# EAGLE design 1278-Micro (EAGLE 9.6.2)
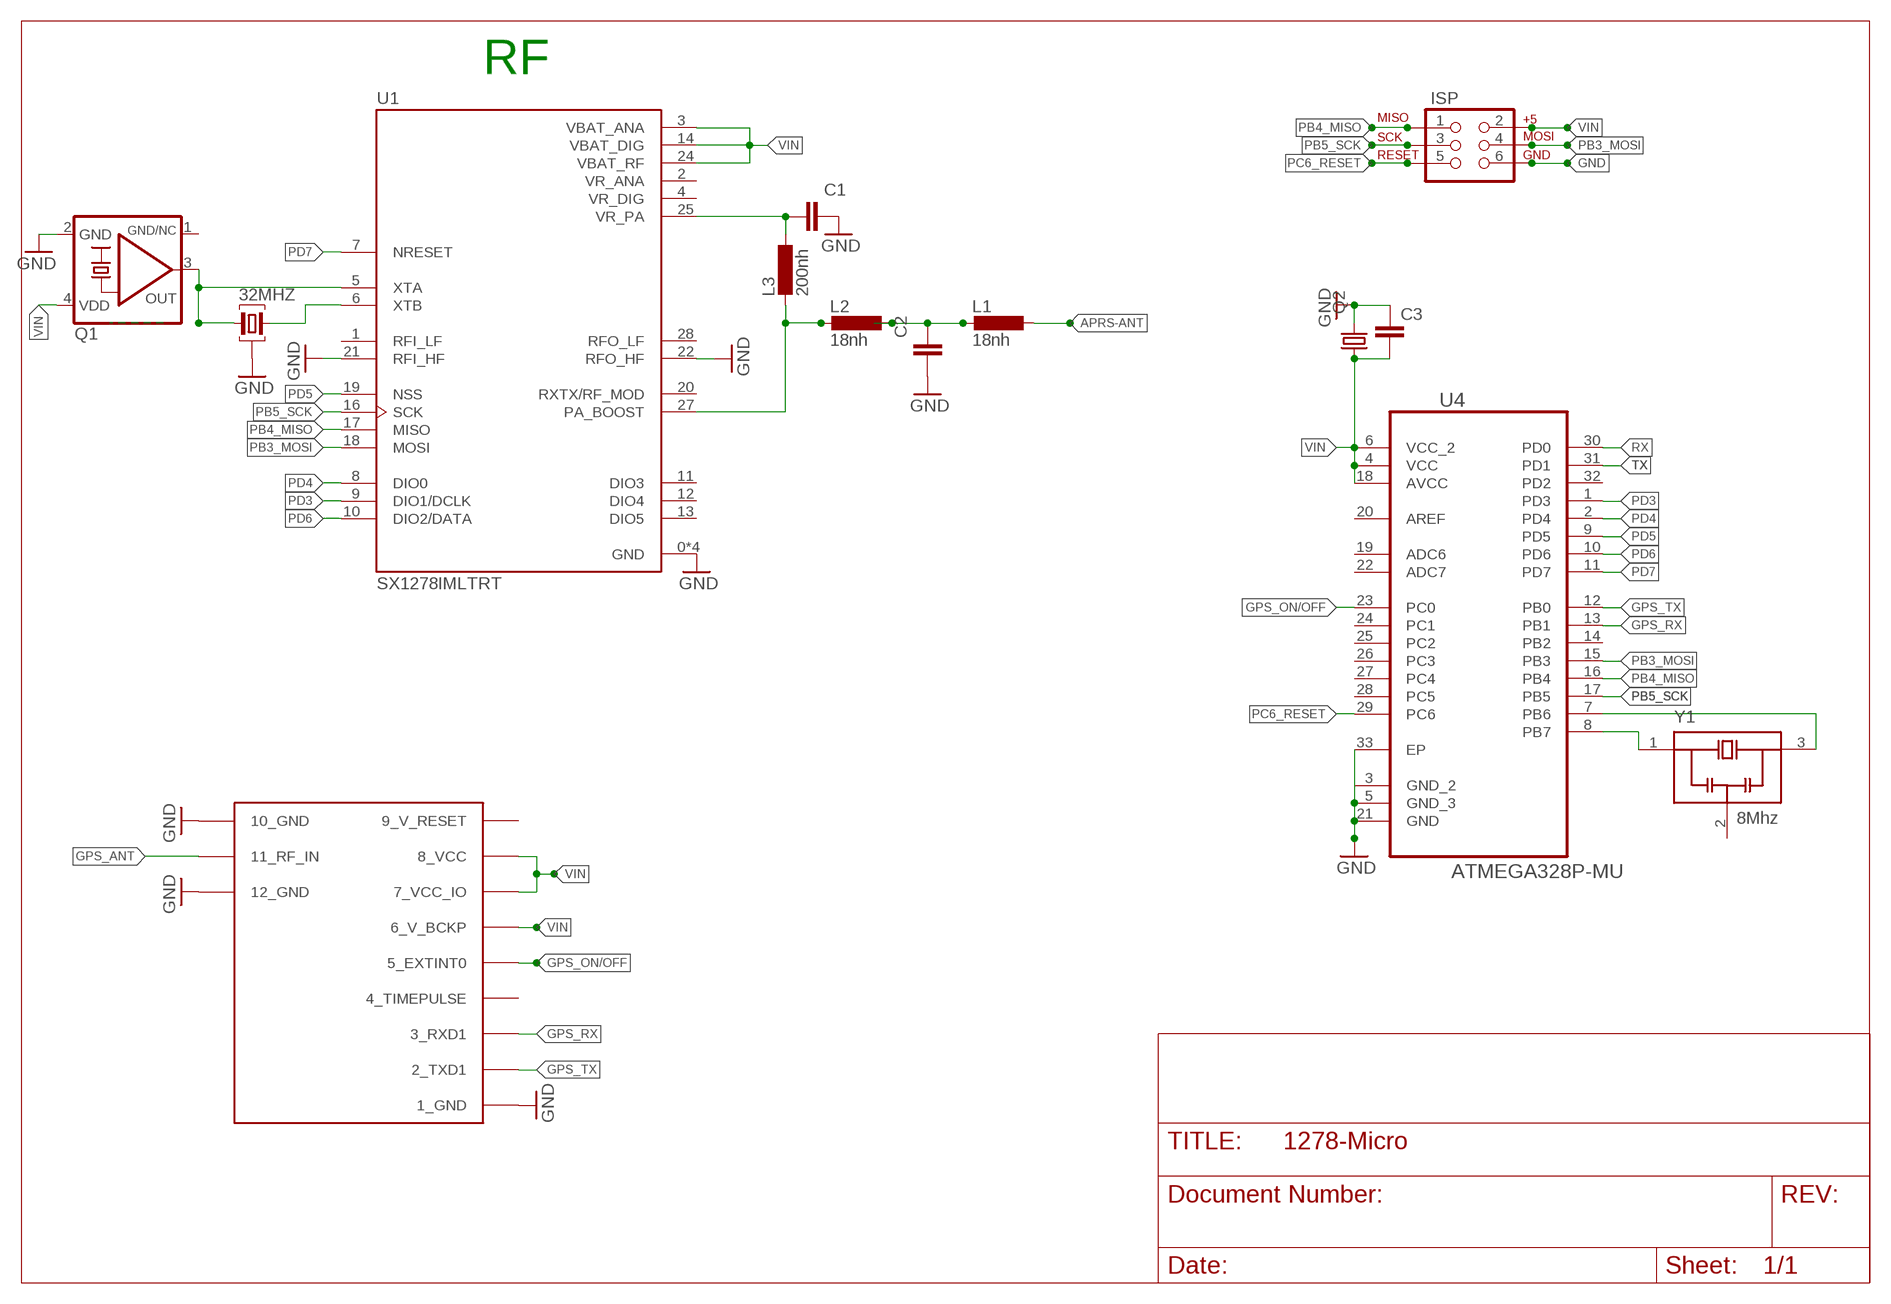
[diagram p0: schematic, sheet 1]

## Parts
32MHZ  16Mhz  ABM8G  [ABM8G]
C1  100nF  C-EUC0603K  [C0603K]
C2  15pF  C-EUC0603K  [C0603K]
C3  C-EUC1808  [C1808]
ISP  AVR_SPI_PRG_6PTH  [2X3]
L1  18nh  L-EUL2012C  [L2012C]
L2  18nh  L-EUL2012C  [L2012C]
L3  200nh  L-EUL2012C  [L2012C]
Q1  TCXO 32Mhz  KXO-TCXO-CMOS-84  [3.2X2.5_KXO-84-TCXO]
Q2  KX-327-NHF  [3.2X1.5]
U1  SX1278IMLTRT  [QFN65P600X600X100-29N]
U4  ATMEGA328P-MU  [QFN50P500X500X100-33N]
U$2  UBLOX_MAX  [UBLOX_MAX]
Y1  8Mhz  CSTCE12M0G15L08-R0  [OSC_CSTCE12M0G15L08-R0]

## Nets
AAA: 32MHZ.1 Q1.3(OUT) U1.5(XTA)
APRS-ANT: L1.1
GND: 32MHZ.2 32MHZ.4 C1.2 C2.1 C3.1 ISP.6 Q1.2(GND) Q2.2 U1.0(GND) U1.15(GND) U1.21(RFI_HF) U1.22(RFO_HF) U1.23(GND) U1.26(GND) U4.3(GND_2) U4.5(GND_3) U4.21(GND) U4.33(EP) U$2.1_GND U$2.10_GND U$2.12_GND
GPS_ANT: U$2.11_RF_IN
GPS_ON/OFF: U4.23(PC0) U$2.5_EXTINT0
GPS_RX: U4.13(PB1) U$2.3_RXD1
GPS_TX: U4.12(PB0) U$2.2_TXD1
N$1: U4.7(PB6) Y1.3(OUT)
N$2: U4.8(PB7) Y1.1(IN)
N$3: C2.2 L1.2 L2.1
N$8: C1.1 L3.1 U1.25(VR_PA)
N$9: L2.2 L3.2 U1.27(PA_BOOST)
N$15: 32MHZ.3 U1.6(XTB)
PB3_MOSI: ISP.4 U1.18(MOSI) U4.15(PB3)
PB4_MISO: ISP.1 U1.17(MISO) U4.16(PB4)
PB5_SCK: ISP.3 U1.16(SCK) U4.17(PB5)
PC6_RESET: ISP.5 U4.29(PC6)
PD3: U1.9(DIO1/DCLK) U4.1(PD3)
PD4: U1.8(DIO0) U4.2(PD4)
PD5: U1.19(NSS) U4.9(PD5)
PD6: U1.10(DIO2/DATA) U4.10(PD6)
PD7: U1.7(NRESET) U4.11(PD7)
RX: U4.30(PD0)
TX: U4.31(PD1)
VIN: C3.2 ISP.2 Q1.4(VDD) Q2.1 U1.3(VBAT_ANA) U1.14(VBAT_DIG) U1.24(VBAT_RF) U4.4(VCC) U4.6(VCC_2) U4.18(AVCC) U$2.6_V_BCKP U$2.7_VCC_IO U$2.8_VCC
Unconnected: U1.1(RFI_LF) U1.11(DIO3) U1.12(DIO4) U1.13(DIO5) U1.20(RXTX/RF_MOD) U1.28(RFO_LF) U4.14(PB2) U4.19(ADC6) U4.20(AREF) U4.22(ADC7) U4.24(PC1) U4.25(PC2) U4.26(PC3) U4.27(PC4) U4.28(PC5) U4.32(PD2) U$2.4_TIMEPULSE

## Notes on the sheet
- RF

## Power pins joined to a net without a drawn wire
9_V_RESET: U$2.9_V_RESET
GND: Y1.2(GND)
GND/NC: Q1.1(GND/NC)
VR_ANA: U1.2(VR_ANA)
VR_DIG: U1.4(VR_DIG)

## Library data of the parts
32MHZ = crystal:ABM8G: CRYSTAL - ABRACON ABM8G Series, 3.2 x 2.5 mm
C1 C2 = rcl:C-EU: CAPACITOR, European symbol; SPICEPREFIX: C
C3 = resistor:C-EU: CAPACITOR, European symbol
ISP = SparkFun:AVR_SPI_PRG_6: AVR ISP 6 Pin This is the reduced ISP connector for AVR programming. Common on Arduino. This footprint will take up less PCB space and can be used with a 10-pin to 6-pin adapter such as SKU: BOB-08508
L1-L3 = resistor:L-EU: INDUCTOR, European symbol
Q1 = crystal-geyer_V1_0:KXO-TCXO-CMOS: TCXO : CMOS - Serie Model Size l/w/h [mm] Frequency Range Frequency Stability Temp. Range [°C] Output AECQ 200 availabel Datasheet KXO-86 KXO-84 KXO-83 KXO-82 2.5/2.0/0.7 3.2/2.5/1.0 5.0/3.2/1.5 7.0/5.0/2.4 13,0 ~ 40,0 MHz 10,0 ~ 40,0 MHz 10,0 ~ 40,0 MHz 10,0 ~ 30,0 MHz ±1,0 … ±2,5ppm ±1,0 …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
Q2 = crystal-geyer_V1_0:KX-327
U1 = SX1278IMLTRT:SX1278IMLTRT; DESCRIPTION: IC RF TxRx Only 802.15.4 LoRa™ 137MHz ~ 525MHz 28-VQFN Exposed Pad; DIGI-KEY_PART_NUMBER: SX1278IMLTRTCT-ND; MF: Semtech; MP: SX1278IMLTRT; PACKAGE: VQFN-28 Semtech
U4 = ava:ATMEGA328P-MU: Programmable Flash; MPN: ATMEGA328P-MU; OC_FARNELL: 1748522; OC_NEWARK: 26R2526; PACKAGE: QFN-32; SUPPLIER: Atmel
U$2 = Max gps:UBLOX_MAX: UBLOX MAX
Y1 = CSTCE12M0G15L08-R0:CSTCE12M0G15L08-R0: 8MHz Ceramic Resonator Built in Capacitor 10pF +/- 0.2% -40C - 125C Surface Mount Check prices; AVAILABILITY: Not in stock; DESCRIPTION: CSTCE Series 12 MHz 3.2 x 1.3 x 0.7 mm Built-in Capacitor SMT Resonator; MF: Murata; MP: CSTCE12M0G15L08-R0; PACKAGE: SMD-3 Murata; PRICE: None

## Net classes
0 default: width 0.203 mm
1 vcc: width 0.152 mm, clearance 0.152 mm

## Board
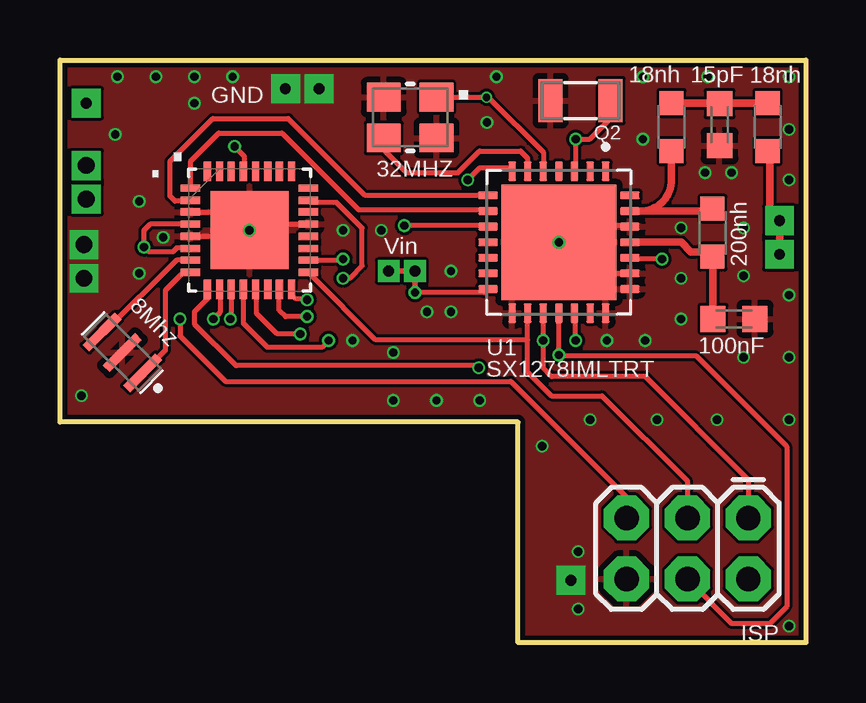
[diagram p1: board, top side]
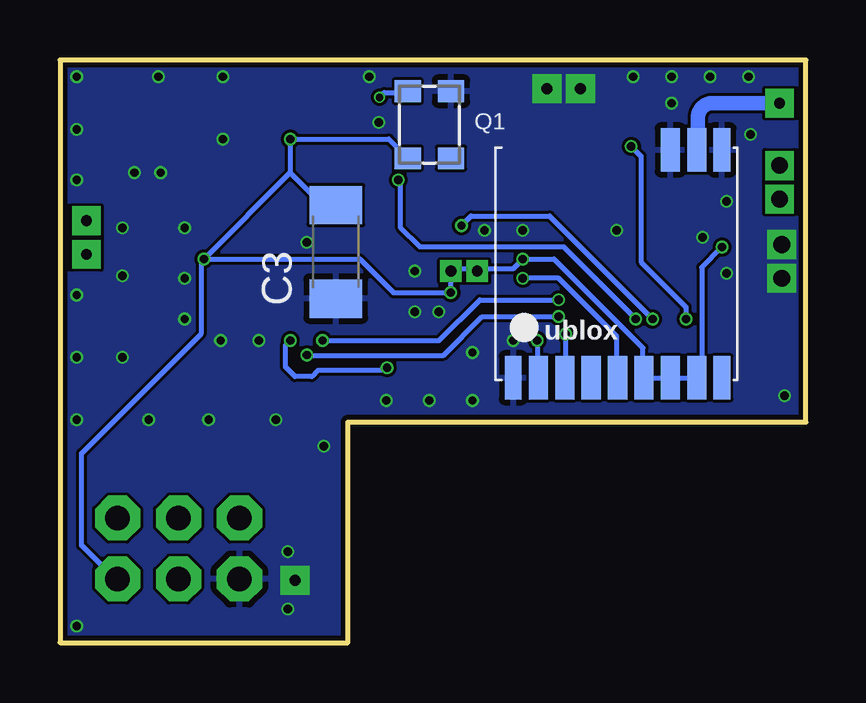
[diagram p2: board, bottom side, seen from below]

Size 31.1 x 24.3 mm. Coordinates in mm from the lower left corner, seen from the top.
Outline: 0,24.3 31.1,24.3 31.1,0 19.1,0 19.1,9.2 0,9.2 0,24.3
Copper layers (1*16): Top 0.035559375mm / dielectric 1.6mm / Bottom 0.035559375mm
Design rules "jlcpcb2layer *": minimum track width 5mil, minimum drill 12mil, track to track 5mil, track to pad 5mil, pad to pad 5mil, via to via 5mil, smd to smd 5mil, copper to edge 8mil, drill to drill 6mil, minimum pad ring 5mil, minimum via ring 3mil, stop-mask expansion 2.5mil, vias tented up to drill 14mil, thermal gap 10mil

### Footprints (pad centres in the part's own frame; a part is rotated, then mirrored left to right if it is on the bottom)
ABM8G = smd 1.4 x 1.2: 1 -1.1,-0.85; 2 1.1,-0.85; 3 1.1,0.85; 4 -1.1,0.85
C0603K = smd 1.05 x 1.08: 1 -0.875,0; 2 0.875,0
C1808 = smd 1.6 x 2.2: 1 -1.95,0; 2 1.95,0
2X3 = drill 1.016 pad 1.88 octagon: 1 0,0; 2 0,2.54; 3 2.54,0; 4 2.54,2.54; 5 5.08,0; 6 5.08,2.54
L2012C = smd 1 x 1: 1 -1,0; 2 1,0
3.2X2.5_KXO-84-TCXO = smd 0.9 x 1.1: 1 -1.4,-0.9; 2 1.4,-0.9; 3 1.4,0.9; 4 -1.4,0.9
3.2X1.5 = smd 1 x 1.8: 1 -1.25,0; 2 1.25,0
QFN65P600X600X100-29N = smd 4.8 x 4.8: 0 0,0 | smd 0.81 x 0.32: 1 -2.955,1.95; 2 -2.955,1.3; 3 -2.955,0.65; 4 -2.955,0; 5 -2.955,-0.65; 6 -2.955,-1.3; 7 -2.955,-1.95; 15 2.955,-1.95; 16 2.955,-1.3; 17 2.955,-0.65; 18 2.955,0; 19 2.955,0.65; 20 2.955,1.3; 21 2.955,1.95 | smd 0.32 x 0.81: 8 -1.95,-2.955; 9 -1.3,-2.955; 10 -0.65,-2.955; 11 0,-2.955; 12 0.65,-2.955; 13 1.3,-2.955; 14 1.95,-2.955; 22 1.95,2.955; 23 1.3,2.955; 24 0.65,2.955; 25 0,2.955; 26 -0.65,2.955; 27 -1.3,2.955; 28 -1.95,2.955
QFN50P500X500X100-33N = smd 0.813 x 0.305: 1 -2.464,1.753; 2 -2.464,1.245; 3 -2.464,0.762; 4 -2.464,0.254; 5 -2.464,-0.254; 6 -2.464,-0.762; 7 -2.464,-1.245; 8 -2.464,-1.753; 17 2.464,-1.753; 18 2.464,-1.245; 19 2.464,-0.762; 20 2.464,-0.254; 21 2.464,0.254; 22 2.464,0.762; 23 2.464,1.245; 24 2.464,1.753 | smd 0.305 x 0.813: 9 -1.753,-2.464; 10 -1.245,-2.464; 11 -0.762,-2.464; 12 -0.254,-2.464; 13 0.254,-2.464; 14 0.762,-2.464; 15 1.245,-2.464; 16 1.753,-2.464; 25 1.753,2.464; 26 1.245,2.464; 27 0.762,2.464; 28 0.254,2.464; 29 -0.254,2.464; 30 -0.762,2.464; 31 -1.245,2.464; 32 -1.753,2.464 | smd 3.251 x 3.251: 33 0,0
UBLOX_MAX = smd 1.8 x 0.7: 1_GND 4.95,-4.4; 9_V_RESET 4.95,4.3; 10_GND -4.55,4.3 | smd 1.8 x 0.8: 2_TXD1 4.95,-3.35; 3_RXD1 4.95,-2.25; 4_TIMEPULSE 4.95,-1.15; 5_EXTINT0 4.95,-0.05; 6_V_BCKP 4.95,1.05; 7_VCC_IO 4.95,2.15; 8_VCC 4.95,3.25; 11_RF_IN -4.55,3.25; 12_GND -4.55,2.15
OSC_CSTCE12M0G15L08-R0 = smd 0.4 x 1.9: 1 -1.2,0; 2 0,0; 3 1.2,0

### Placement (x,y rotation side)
32MHZ  14.6,21.9 180 top
C1  28.1,13.5 0 top
C2  27.5,21.6 90 top
C3  19.6,16.3 90 bottom
ISP  28.7,5.2 180 top
L1  29.5,21.5 90 top
L2  25.5,21.5 270 top
L3  27.2,17.1 90 top
Q1  15.7,21.6 90 bottom
Q2  21.7,22.6 180 top
U1  20.8,16.7 270 top
U4  7.9,17.2 0 top
U$2  7.8,16 270 bottom
Y1  2.6,12.1 135 top

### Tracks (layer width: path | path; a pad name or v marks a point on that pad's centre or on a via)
AAA  (via drill 0.3)
  Top 0.203: 32MHZ.1 v17.78,22.75 | v17.78,22.75 17.85,22.75 20.15,20.45 U1.5 | v17.78,22.74 v17.78,22.75
  Bottom 0.203: v17.78,22.74 17.58,22.94 16.66,22.94 Q1.3
APRS-ANT  (via drill 0.45 pad 1.2)
  Top 0.305: v30,16.2 v30,17.6 arc-90 29.6,18 29.6,20.4 L1.1
GND  (via drill 0.35, 0.45 pad 1.2, 0.7 pad 1.2)
  Top 0.203: U4.5 6.75,16.95 6.8,16.9 7.1,16.9 | 7.1,16.9 7.89,16.9 | 7.89,16.9 8.6,16.9 9.15,17.45 U4.21 | U4.3 6.74,17.96 7.1,17.6 7.1,16.9 | 7.89,16.9 7.89,17.14 U4.33 | 22.2,17.29 21.3,17.29 20.84,16.84 U1.0 | U1.26 23.71,17.39 22.2,17.39 22.2,17.29 | U1.23 22.6,15.4 22.2,15.8 22.2,17.29
  other vias: 13.9,12.1 15.3,13.8 21.6,1.4 4.3,16.9 13.9,10.1 1,16.6 1,15.2 2.3,21.2 2.4,23.6 7.2,23.6 15.7,10.1 17.5,10.1 21.6,3.8 30.4,0.7 3.3,18.4 17.8,21.7 18.2,23.6 27,23.6 30.4,23.6 24.4,12.6 22.8,12.6 30.4,19.3 30.4,21.4 28,19.6 26.9,19.6 24.3,21 25.9,17.3 25.9,13.5 28.5,17.3 28.5,15.3 30.4,14.5 30.4,11.9 28.5,11.9 25.9,15.2 12.2,12.6 22.1,9.3 24.9,9.3 27.4,9.3 20.1,8.2 16.3,13.8 5.6,23.6 4,23.6 5.6,22.5 20.8,16.7 11.8,17.2 13.4,17.2 30.4,9.3 10.8,23.1 9.4,23.1 16.3,15.5 0.9,10.3 3.3,15.4 24.3,23.6 7.9,17.2 21.3,2.6
  pour Top: -12.19,36.02 41.75,36.02 41.75,-7.09 -12.19,-7.09
  pour Bottom: -12.19,36.02 41.75,36.02 41.75,-7.09 -12.19,-7.09
GPS_ANT  (via drill 0.45 pad 1.2)
  Bottom 0.203: 4.5,20.6 arc90 U$2.11_RF_IN
  Bottom 0.61: v1.1,22.5 3.9,22.5 arc-90 4.5,21.9 4.5,20.6
GPS_ON/OFF  (via drill 0.35)
  Top 0.203: U4.23 10.45,18.36 11.54,18.36 12.6,17.29 12.6,15.72 12.09,15.2 v11.8,15.2
  Bottom 0.203: v11.8,15.2 10.31,15.2 7.89,12.77 7.89,11.2 U$2.5_EXTINT0
GPS_RX  (via drill 0.35)
  Top 0.203: v10.02,12.87 9.06,12.87 8.19,13.74 8.19,14.7 U4.13
  Bottom 0.203: U$2.3_RXD1 10.02,11.08 v10.02,12.87
GPS_TX  (via drill 0.35)
  Top 0.203: U4.12 7.64,14.73 7.64,13.34 8.66,12.32 10.92,12.32 v11.2,12.6
  Bottom 0.203: v11.2,12.6 v11.19,12.59 11.19,11.09 U$2.2_TXD1
N$1
  Top 0.203: U4.7 4.86,15.96 1.85,12.95 Y1.3
N$2
  Top 0.203: Y1.1 4.4,12.2 4.4,14.7 5.15,15.45 U4.8
N$3
  Top 0.203: 27.15,22.5 27.18,22.48 C2.2 27.53,22.5
  Top 0.305: L2.1 27.15,22.5 | L1.2 27.53,22.5
N$8
  Top 0.203: L3.1 27.22,16.07
  Top 0.305: U1.25 25.9,16.7 26.3,16.3 27,16.3 L3.1 | 27.22,16.07 C1.1
N$9
  Top 0.203: L3.2 27.25,18.1 27.35,18
  Top 0.305: 27.35,18 24.2,18 | 24.2,18 U1.27 | L2.2 25.5,19.3 arc-90 24.2,18
N$10  (via drill 0.7 pad 1.2)
  other vias: 1.1,19.9
N$11  (via drill 0.7 pad 1.2)
  other vias: 1.1,18.5
N$15
  Top 0.203: 32MHZ.3 13.5,20.55 14.45,19.6 16.6,19.6 17.5,20.5 19.2,20.5 19.5,20.2 U1.6
PB3_MOSI  (via drill 0.35)
  Top 0.203: U1.18 v20.8,12 20.84,11.96 26.53,11.96 30.3,8.19 30.3,1.5 29.6,0.8 28.02,0.8 ISP.4 | v10.3,13.6 9.4,13.6 9.14,13.86 U4.15
  Bottom 0.203: v20.8,12 20.78,11.98 15.12,11.98 13.5,13.6 v10.3,13.6
PB4_MISO  (via drill 0.35)
  Top 0.203: U1.17 v20.15,12.6 20.15,11.45 20.5,11.1 24.4,11.1 28.7,6.8 ISP.1 | v10.3,14.3 10.26,14.34 9.85,14.34 9.65,14.54 U4.16
  Bottom 0.203: v20.15,12.6 15.3,12.6 13.6,14.3 v10.3,14.3
PB5_SCK
  Top 0.203: 19.5,12.63 19.5,11.3 20.5,10.3 22.6,10.3 26.16,6.74 ISP.3 | 19.5,12.63 U1.16 | 19.5,12.63 13.17,12.63 10.48,15.31 U4.17
PC6_RESET  (via drill 0.35)
  Top 0.203: U4.29 7.68,19.7 7.68,20.29 v7.28,20.69 | v5,13.5 5,12.8 6.9,10.9 18.8,10.9 23.62,6.08 ISP.5
  Bottom 0.203: v7.28,20.69 6.88,20.29 6.88,15.88 5,14 v5,13.5
PD3
  Top 0.203: U1.9 17.79,18.06 12.46,18.06 9.26,21.25 6.62,21.25 5.45,20.08 5.45,18.97 U4.1
PD4
  Top 0.203: U4.2 5.4,18.41 4.79,18.41 4.59,18.62 4.59,20.08 6.36,21.86 9.51,21.86 12.7,18.66 17.79,18.66 U1.8
PD5  (via drill 0.35)
  Top 0.203: 21.45,13.48 21.45,13.64 U1.19 21.5,13.7 v21.5,12.6 | U4.9 6.15,14.35 5.6,13.8 5.6,13.3 7.34,11.56 17.37,11.56 v17.46,11.47
  Bottom 0.203: v17.46,11.47 17.56,11.37 20.33,11.37 20.6,11.1 21.3,11.1 21.7,11.5 21.7,12.4 v21.5,12.6
PD6  (via drill 0.35)
  Top 0.203: U1.10 17.8,17.39 v14.36,17.39 | U4.10 6.67,14.72 6.67,13.77 v6.4,13.5
  Bottom 0.203: v14.36,17.39 13.96,17.79 10.69,17.79 v6.4,13.5
PD7  (via drill 0.35)
  Top 0.203: 7.13,14.65 7.14,14.66 U4.11 7.14,13.54 v7.1,13.5 | 18.81,19.73 18.8,19.71 U1.7 18.89,19.7 18.79,19.8 17.5,19.8 v17,19.3
  Bottom 0.203: v17,19.3 16.9,19.2 16.9,17.3 16.1,16.5 10.1,16.5 v7.1,13.5
VIN  (via drill 0.35, 0.45 pad 0.9)
  Top 0.203: U1.3 21.5,19.71 v21.5,21 22.1,21 22.95,21.85 Q2.1 | U1.14 17.69,14.6 v14.8,14.6 | v25.1,16 23.8,16 U1.24 | U4.18 11.75,15.96 v11.8,16 | 5.4,16.4 U4.6 5.38,16.44 5.36,16.46 4.86,16.46 4.7,16.3 3.7,16.3 v3.5,16.5 3.5,17.2 3.75,17.45 U4.4 | v14.8,14.6 14.8,15.4 14.7,15.5 v13.7,15.5 v14.8,15.5 v14.8,14.6
  Bottom 0.203: v25.1,16 18.6,16 17.2,14.6 v14.8,14.6 v14.8,15.5 14.7,15.6 12.2,15.6 v11.8,16 10.5,16 6.8,12.3 6.8,11.1 U$2.6_V_BCKP U$2.7_VCC_IO U$2.8_VCC 4.35,11.25 4.35,15.65 v3.5,16.5 | 21.5,19.6 v21.5,21 17.4,21 Q1.4 | 21.5,19.6 v25.1,16 | v25.1,16 25.2,15.9 25.2,12.9 30.2,7.9 30.2,4.06 28.8,2.66 ISP.2 | 21.5,19.6 20.15,18.25 C3.2

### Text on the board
tPlace: .
tNames: GND | Vin

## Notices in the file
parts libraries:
crystal-geyer_V1_0: Copyright: Geyer-Electronic
